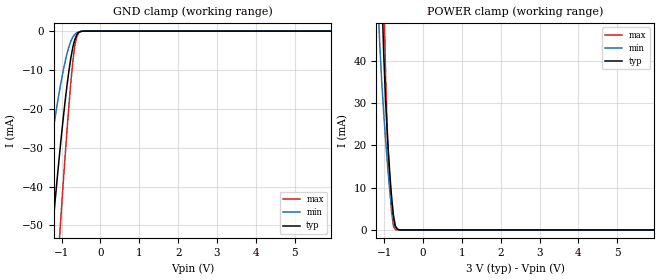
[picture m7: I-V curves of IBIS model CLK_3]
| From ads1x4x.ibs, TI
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|   CLK 3.0V model
[Model]   CLK_3
Model_type   Input
| Signals   CLK
Vinl =  0.45V
Vinh =  1.20V
| variable   typ   min   max
C_comp   7.269pF   8.099pF   6.450pF
[Temperature Range]   40.0   105.0   -40.0
[Voltage range]   5.0V   4.75V   5.25V
[power clamp reference] 3.0V   2.7V   3.3V
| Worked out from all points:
|   GND clamp passes 1 mA (typ) near -0.61 V on its own axis
|   POWER clamp passes 1 mA (typ) near -0.71 V on its own axis
[GND Clamp]
|   Voltage   I(typ)   I(min)   I(max)
-3V       -286.5mA   -193.8mA   -373.3mA
-1.56V    -90.61mA   -51.46mA   -134.9mA
-1.26V    -54.21mA   -28.5mA    -85.83mA
-1.21V    -48.53mA   -25.08mA   -77.82mA
-1.06V    -32.41mA   -15.7mA    -54.31mA
-1.01V    -27.41mA   -12.89mA   -46.74mA
-859.9mV  -13.92mA   -5.781mA   -25.45mA
-759.9mV  -6.818mA   -2.546mA   -12.99mA
-659.9mV  -2.173mA   -821.9uA   -3.806mA
-609.9mV  -946.5uA   -430.4uA   -1.447mA
-409.9mV  -7.591uA   -12.33uA   -3.615uA
5.94V     0A         0A         0A
[POWER Clamp]
|   Voltage   I(typ)   I(min)   I(max)
-3V       1.061A     857.9mA    1.359A
-1.16V    95.66mA    54.5mA     139.3mA
-1.11V    75mA       43.6mA     110mA
-1.06V    56.68mA    34.93mA    82.2mA
-1.01V    41.63mA    27.65mA    56.99mA
-959.9mV  30.21mA    21.16mA    36.19mA
-909.9mV  21.47mA    15.21mA    21.47mA
-859.9mV  14.23mA    9.855mA    11.58mA
-809.9mV  8.107mA    5.381mA    4.582mA
-759.9mV  3.468mA    2.25mA     908.5uA
-709.9mV  950.3uA    689.5uA    94.99uA
5.94V     0A         0A         0A
